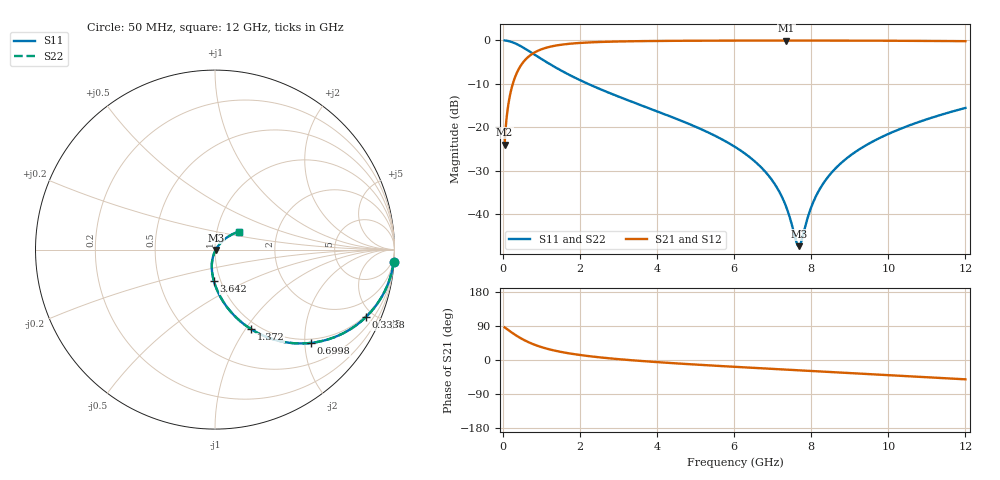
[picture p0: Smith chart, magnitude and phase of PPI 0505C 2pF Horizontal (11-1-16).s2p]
# MHz S MA R 50
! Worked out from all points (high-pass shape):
!   1601 points, 50 MHz to 12 GHz, reference 50 ohm
!   highest |S21| = -0.04 dB at 7.354 GHz (marker M1); lowest = -24.0 dB at 50 MHz (marker M2)
!   |S21| within 3 dB of the highest: 777.4 MHz to end of sweep
!   lowest |S11| = -47.3 dB at 7.676 GHz (marker M3), VSWR 1.01, Z = 50.4 - j0.211 ohm
!   |S11| at or under -10 dB: 2.214 GHz to end of sweep
!   |S22| runs from -47.3 to 0.0 dB; largest |S21 - S12| = 0
!   S11 on the Smith chart (normalised r, x): 50 MHz: 1, -30; 333.8 MHz: 0.91, -4.49; 699.8 MHz: 0.91, -2.13; 1.372 GHz: 0.91, -1.07; 3.642 GHz: 0.93, -0.34; 12 GHz: 1.28, +0.26
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50  0.998 -3.8  0.06342 86.2  0.06342 86.2  0.998 -3.8
176.9688  0.9755 -13.3  0.2195 76.7  0.2195 76.7  0.9755 -13.3
333.8125  0.9202 -24.2  0.3909 65.7  0.3909 65.7  0.9202 -24.2
490.6562  0.8474 -33.8  0.5299 56.2  0.5299 56.2  0.8474 -33.8
699.7812  0.7447 -44.3  0.6661 45.6  0.6661 45.6  0.7447 -44.3
1013.469  0.6078 -56.1  0.7924 33.8  0.7924 33.8  0.6078 -56.1
1371.969  0.4882 -65.5  0.8707 24.3  0.8707 24.3  0.4882 -65.5
2044.156  0.3425 -77.0  0.9371 12.7  0.9371 12.7  0.3425 -77.0
3642.469  0.1757 -92.0  0.9812 -3.0  0.9812 -3.0  0.1757 -92.0
4038.312  0.1508 -94.6  0.9852 -5.8  0.9852 -5.8  0.1508 -94.6
6025  0.0596 -104.5  0.9941 -18.1  0.9941 -18.1  0.0596 -104.5
6854.031  0.02931 -104.8  0.9951 -22.7  0.9951 -22.7  0.02931 -104.8
7137.844  0.01942 -102.0  0.9953 -24.2  0.9953 -24.2  0.01942 -102.0
7354.438  0.01212 -95.2  0.9953 -25.4  0.9953 -25.4  0.01212 -95.2
7608.375  0.004949 -57.1  0.9952 -26.8  0.9952 -26.8  0.004949 -57.1
7675.594  0.004298 -29.2  0.9952 -27.1  0.9952 -27.1  0.004298 -29.2
7750.281  0.004969 2.0  0.9952 -27.5  0.9952 -27.5  0.004969 2.0
8019.156  0.01264 40.5  0.995 -29.0  0.995 -29.0  0.01264 40.5
8317.906  0.02277 47.9  0.9947 -30.6  0.9947 -30.6  0.02277 47.9
8728.688  0.03715 49.9  0.9941 -32.8  0.9941 -32.8  0.03715 49.9
10013.31  0.08441 46.7  0.9906 -39.8  0.9906 -39.8  0.08441 46.7
12000  0.1672 36.9  0.9791 -51.0  0.9791 -51.0  0.1672 36.9
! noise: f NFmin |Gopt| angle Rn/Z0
50  0.0008944  0.9506  1.628  0.004061
1372  0.005538  0.7557  6.23  0.004568
2701  0.008628  0.7008  10.7  0.005598
4031  0.01134  0.6683  15.19  0.006456
5360  0.01389  0.647  19.63  0.007252
6682  0.01635  0.633  23.96  0.008034
8012  0.01883  0.6243  28.21  0.008848
9341  0.02136  0.6201  32.35  0.009719
1.067e+04  0.02399  0.6196  36.37  0.01068
1.2e+04  0.02676  0.6223  40.26  0.01175
